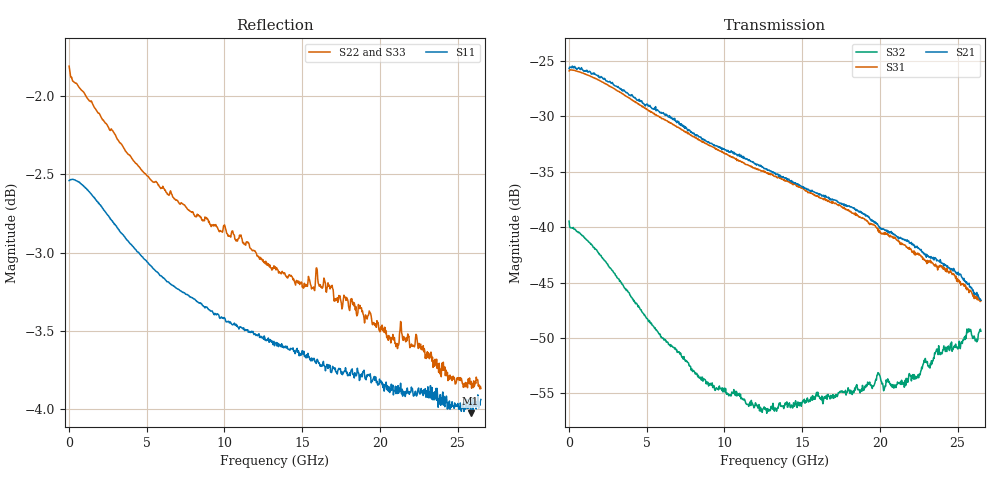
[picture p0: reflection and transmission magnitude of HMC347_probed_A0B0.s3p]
! Hittite Microwave Corporation
! 20 Alpha Road
! Chelmsford, MA 01824
! http://www.hittite.com
! Tel: 978-250-3343
! Fax: 978-250-3373
! Device:  HMC347
! Description: GaAs MMIC SPDT Non-Reflective Switch
! Frequency:  DC -  20.00 GHz
! Package:  DIE
! Ports:  3 RF, 2 DC
!  Pad  1 = RF1 = Port 2
!  Pad  2 = Control A [Alternate]
!  Pad  3 = Control B [Alternate]
!  Pad  4 = RFC = Port 1
!  Pad  5 = Control A [Alternate]
!  Pad  6 = Control B [Alternate]
!  Pad  7 = RF2 = Port 3
!  Pad  8 = Control A
!  Pad  9 = Control B
!  Pad 10 = Control A [Alternate]
! Control:  -5 Volt control voltage
!  Low  = 0 =  0 V
!  High = 1 = -5 V
! State:  Both Low, Undefined
! Voltages:  VA =  0.0 Volts
!  VB =  0.0 Volts
! Data:  The device was measured using G-S-G Probes at the chip ports.
!  Data was collected using an calibrated 3 port network analyzer.
!  The reference plane is the pads on the switch chip.
! Misc:  Die 64601
!  Lot GB01, Tested Unit 3
! Date Measured:  2010-03-11
! Date:  2010-03-15
! Note:
!  Hittite supplies this data as a sample of measured data at the package pin for
!  for this package product.  Your particular data for this product may vary.
!  Data was taken at 25 degrees C.
!  Hittite reserves the right to change this data at anytime.
!S3P File: Measurements: <S11,S12,S13>,
!  <S21,S22,S23>,
!  <S31,S32,S33>:
# Hz S  dB  R 50
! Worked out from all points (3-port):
!   801 points, 10 MHz to 26.5 GHz, reference 50 ohm
!   strongest paths, dB at 10 MHz, 6.633 GHz, 13.26 GHz, 19.88 GHz, 26.5 GHz:
!     S21: -25.7, -30.1, -35.1, -39.8, -46.6
!     S31: -25.9, -30.6, -35.4, -40.4, -46.7
!     S32: -39.4, -50.7, -56.3, -53.1, -49.4
!   lowest |S11| = -4.0 dB at 25.84 GHz (marker M1), VSWR 4.39, Z = 11.9 + j10.1 ohm
!   |S11| at or under -10 dB: nowhere
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1e7  -2.54 -179.9  -25.90 -0.3  -25.85 -0.4
     -25.67 0.5  -1.81 -179.9  -39.70 2.4
     -25.88 -1.8  -39.45 -8.4  -1.71 179.9
1.268275e9  -2.61 177.3  -26.37 -17.4  -26.37 -18.1
            -25.98 -17.2  -2.02 174.6  -40.60 -37.8
            -26.29 -18.0  -41.34 -37.6  -1.81 174.6
8.387462e9  -3.32 169.6  -32.16 -73.4  -32.22 -74.4
            -31.83 -74.1  -2.76 152.5  -53.13 -140.2
            -32.16 -74.3  -53.60 -141.1  -2.54 152.5
1.3255e10  -3.58 165.8  -35.45 -94.9  -35.51 -95.8
           -35.09 -95.2  -3.09 138.2  -56.03 178.2
           -35.42 -96.5  -56.32 178.3  -2.88 138.5
1.885101e10  -3.79 161.8  -38.91 -121.5  -39.19 -123.2
             -38.74 -121.8  -3.38 121.4  -54.93 131.2
             -39.16 -124.3  -54.81 128.9  -3.18 122.5
1.98775e10  -3.85 161.0  -39.95 -126.9  -40.25 -128.7
            -39.81 -126.4  -3.45 118.2  -53.52 125.6
            -40.35 -129.9  -53.14 123.9  -3.24 119.5
2.024174e10  -3.84 160.7  -40.28 -127.1  -40.57 -127.9
             -40.19 -126.2  -3.49 117.3  -54.70 123.0
             -40.61 -128.4  -54.78 119.6  -3.26 118.4
2.150001e10  -3.89 159.4  -41.21 -131.8  -41.61 -133.9
             -41.07 -130.6  -3.56 113.1  -54.55 119.8
             -41.57 -133.8  -54.20 115.4  -3.30 114.5
2.583775e10  -4.03 156.0  -45.68 -151.2  -45.68 -147.6
             -45.37 -149.9  -3.83 99.6  -49.79 84.5
             -45.70 -148.7  -49.25 77.6  -3.44 101.3
2.65e10  -3.94 155.7  -46.70 -152.1  -46.60 -147.2
         -46.60 -150.2  -3.87 98.0  -49.51 81.7
         -46.65 -147.2  -49.40 78.1  -3.46 99.4
